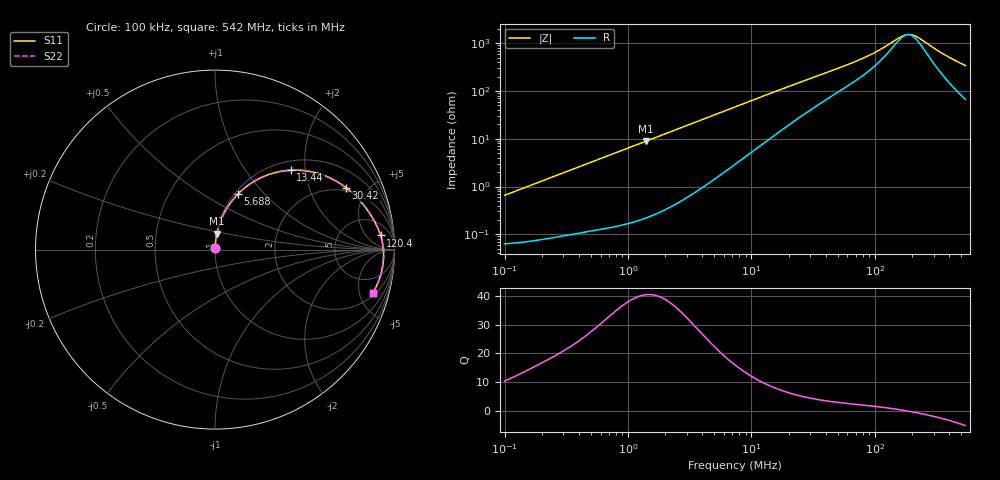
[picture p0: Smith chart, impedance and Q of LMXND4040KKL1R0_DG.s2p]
! LMXND4040KKL1R0_DG  S-PARAMETER MODEL  ( General Type )
! Model Generated by TAIYO YUDEN Corporation (http://www.ty-top.com)
! Version 1.0
! TAIYO YUDEN Control No. 191023NI43SB-FBB
! Copyright(c) 2019 TAIYO YUDEN CO.,LTD. All Rights Reserved.
! Product Description (link to TY-COMPAS)
! https://ds.yuden.co.jp/TYCOMPAS/or/detail?pn=LMXND4040KKL1R0NDG&u=M
! Products Name : Inductors
! Characteristics :
!  Inductance : 1.0 uH , SRF(min) : 116 MHz , DC Resistance(max) : 0.0672 Ohm
!  Rated Current : Saturation :2000 mA , Temp Rise : 1900 mA
!  Case Size : 4.0 x 4.0 / 0.157 x 0.157 [mm/inch] , Thickness : 1 / 0.039 [mm/inch]
!  (Conditions: Temperature = 25 degC , DC Bias Current/Voltage = 0A / 0V)
! External Node Assignments :
!  1  o---GGG---o  2
! GND o---------o GND
! Frequency Range : 0.1MHz  -  542.002916MHz  [ 402 STEP ]
# MHz S RI R 50
! Freq[MHz].  S11 Real  S11 Imag  S21 Real  S21 Imag  S12 Real  S12 Imag  S22 Real  S22 Imag
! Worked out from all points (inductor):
!   401 points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, 100 kHz to 542 MHz, reference 50 ohm
!   read as one part in series: L = 1.03 uH near 104.4 kHz
!   highest Q = 40.4 at 1.407 MHz (marker M1), where L = 1.01 uH
!   self-resonance near 184.6 MHz
!   S11 on the Smith chart (normalised r, x): 100 kHz: 1.00, +0.01; 5.688 MHz: 1.04, +0.72; 13.44 MHz: 1.18, +1.67; 30.42 MHz: 1.82, +3.61; 120.4 MHz: 12, +13; 542 MHz: 2.32, -6.69
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0.1  0.00067 0.00651  0.9993 -0.00651  0.9993 -0.00651  0.00067 0.00651
0.422129  0.0018 0.0269  0.9982 -0.0269  0.9982 -0.0269  0.0018 0.0269
1.406713  0.01 0.088  0.99 -0.088  0.99 -0.088  0.01 0.088
1.78193  0.0153 0.1107  0.9847 -0.1107  0.9847 -0.1107  0.0153 0.1107
3.46957  0.0522 0.2062  0.9478 -0.2062  0.9478 -0.2062  0.0522 0.2062
5.688277  0.126 0.3079  0.874 -0.3079  0.874 -0.3079  0.126 0.3079
7.362085  0.1919 0.3638  0.8081 -0.3638  0.8081 -0.3638  0.1919 0.3638
13.43943  0.4228 0.4424  0.5772 -0.4424  0.5772 -0.4424  0.4228 0.4424
19.36761  0.579 0.4232  0.421 -0.4232  0.421 -0.4232  0.579 0.4232
30.41663  0.731 0.3445  0.269 -0.3445  0.269 -0.3445  0.731 0.3445
31.0775  0.7367 0.34  0.2633 -0.34  0.2633 -0.34  0.7367 0.34
44.78588  0.8156 0.2636  0.1844 -0.2636  0.1844 -0.2636  0.8156 0.2636
70.33577  0.8782 0.176  0.1218 -0.176  0.1218 -0.176  0.8782 0.176
93.01035  0.9048 0.1252  0.0952 -0.1252  0.0952 -0.1252  0.9048 0.1252
120.3792  0.9226 0.0788  0.0774 -0.0788  0.0774 -0.0788  0.9226 0.0788
131.1872  0.9272 0.0632  0.0728 -0.0632  0.0728 -0.0632  0.9272 0.0632
169.7897  0.9365 0.0158  0.0635 -0.0158  0.0635 -0.0158  0.9365 0.0158
185.034  0.9382 -0.000432  0.0618 0.000432  0.0618 0.000432  0.9382 -0.000432
201.6468  0.9392 -0.0169  0.0608 0.0169  0.0608 0.0169  0.9392 -0.0169
229.4043  0.9392 -0.0422  0.0608 0.0422  0.0608 0.0422  0.9392 -0.0422
376.1028  0.9209 -0.1485  0.0791 0.1485  0.0791 0.1485  0.9209 -0.1485
542.0029  0.8808 -0.2398  0.1192 0.2398  0.1192 0.2398  0.8808 -0.2398
